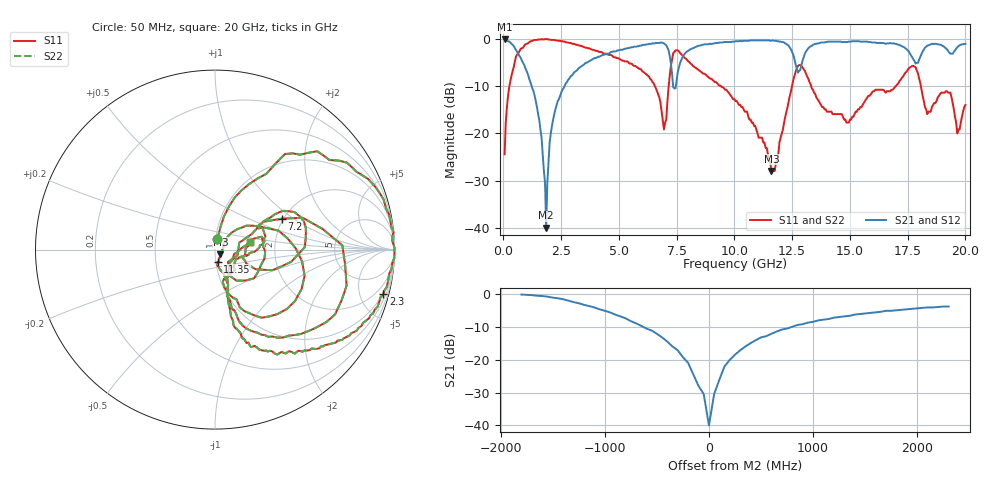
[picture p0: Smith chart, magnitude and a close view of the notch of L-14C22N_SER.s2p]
# MHZ S MA R 50
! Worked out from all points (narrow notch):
!   400 points, 50 MHz to 20 GHz, reference 50 ohm
!   highest |S21| = -0.09 dB at 50 MHz (marker M1); lowest = -40.0 dB at 1.85 GHz (marker M2)
!   notch at M2: 38.6 dB deep, 389 MHz wide at half that depth
!   lowest |S11| = -28.0 dB at 11.6 GHz (marker M3), VSWR 1.08, Z = 53 - j2.81 ohm
!   |S11| at or under -10 dB: 9.419 GHz to 12.5 GHz (3.077 GHz wide, 28.1 % of centre); 13.32 GHz to 16.98 GHz (3.659 GHz wide, 24.1 % of centre); 18.07 GHz to end of sweep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
!   |S22| runs from -28.0 to 0.0 dB; largest |S21 - S12| = 0
!   S11 on the Smith chart (normalised r, x): 50 MHz: 1.02, +0.12; 2.3 GHz: 0.89, -7.54; 7.2 GHz: 1.96, +0.81; 11.35 GHz: 1.02, -0.14; 20 GHz: 1.48, +0.14
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50  0.06 77.6  0.99 -2.5  0.99 -2.5  0.06 77.6
550  0.66 53.8  0.76 -39.6  0.76 -39.6  0.66 53.8
1350  0.98 16.6  0.25 -75.9  0.25 -75.9  0.98 16.6
1650  1 5.6  0.09 -82.4  0.09 -82.4  1 5.6
1850  1 -1.2  0.01 43.0  0.01 43.0  1 -1.2
2000  0.99 -6.1  0.08 75.9  0.08 75.9  0.99 -6.1
2300  0.97 -14.9  0.2 72.6  0.2 72.6  0.97 -14.9
3400  0.84 -38.4  0.52 51.6  0.52 51.6  0.84 -38.4
6700  0.26 -74.0  0.91 3.2  0.91 3.2  0.26 -74.0
6950  0.11 -41.3  0.9 -7.8  0.9 -7.8  0.11 -41.3
7200  0.41 24.9  0.66 -29.5  0.66 -29.5  0.41 24.9
7400  0.73 -6.7  0.3 -1.9  0.3 -1.9  0.73 -6.7
7750  0.67 -44.6  0.64 29.0  0.64 29.0  0.67 -44.6
10050  0.22 -71.8  0.95 -1.2  0.95 -1.2  0.22 -71.8
11350  0.07 -78.2  0.97 -13.1  0.97 -13.1  0.07 -78.2
11600  0.04 -41.5  0.96 -16.0  0.96 -16.0  0.04 -41.5
12750  0.52 -16.3  0.44 -21.8  0.44 -21.8  0.52 -16.3
13350  0.3 -66.6  0.85 -2.2  0.85 -2.2  0.3 -66.6
14850  0.13 -33.0  0.93 -20.7  0.93 -20.7  0.13 -33.0
16700  0.28 28.1  0.9 -35.0  0.9 -35.0  0.28 28.1
19650  0.1 -44.0  0.82 -31.9  0.82 -31.9  0.1 -44.0
20000  0.2 13.0  0.89 -39.3  0.89 -39.3  0.2 13.0
